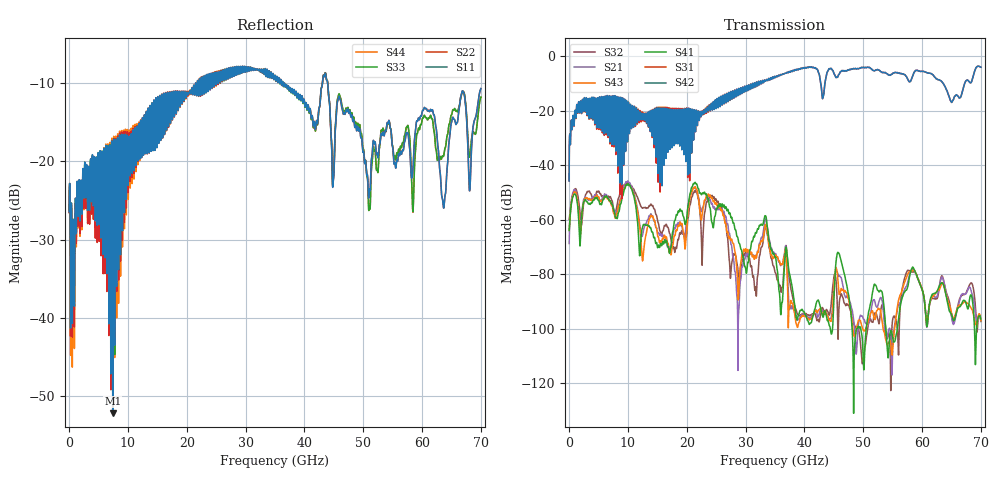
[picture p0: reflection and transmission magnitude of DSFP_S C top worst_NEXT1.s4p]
! AWR Design Environment (8415) Wed Jan 09 11:08:23 2019
! Document = 'DSFP_S'
! nPorts: 4, nXvals: 7001
# HZ S DB R 50
!Freq DBS11 AngS11 DBS12 AngS12 DBS13 AngS13 DBS14 AngS14
!	DBS21 AngS21 DBS22 AngS22 DBS23 AngS23 DBS24 AngS24
!	DBS31 AngS31 DBS32 AngS32 DBS33 AngS33 DBS34 AngS34
!	DBS41 AngS41 DBS42 AngS42 DBS43 AngS43 DBS44 AngS44
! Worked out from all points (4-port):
!   7000 points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, 10 MHz to 70 GHz, reference 50 ohm
!   strongest paths, dB at 10 MHz, 17.51 GHz, 35.01 GHz, 52.51 GHz, 70 GHz:
!     S42: -45.8, -29.4, -7.6, -5.0, -4.0
!     S31: -45.8, -28.1, -7.6, -5.0, -4.0
!     S41: -64.0, -66.0, -73.7, -86.0, -96.5
!     S43: -63.7, -70.0, -73.7, -92.7, -97.0
!     S21: -68.8, -66.5, -72.7, -91.4, -97.0
!     S32: -59.8, -68.3, -79.3, -96.8, -97.4
!   lowest |S11| = -52.2 dB at 7.42 GHz (marker M1), VSWR 1.00, Z = 50 + j0.24 ohm
!   |S11| at or under -10 dB: start of sweep to 21.5 GHz; 36.64 GHz to 43.07 GHz (6.432 GHz wide, 16.1 % of centre); 43.96 GHz to end of sweep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
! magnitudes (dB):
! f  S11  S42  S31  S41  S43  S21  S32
! 10 MHz  -26.4  -45.8  -45.8  -64.0  -63.7  -68.8  -59.8
! 7.42 GHz  -52.2  -15.2  -15.4  -55.0  -55.9  -55.0  -54.2
! 17.05 GHz  -11.2  -21.9  -21.3  -72.4  -72.0  -72.1  -64.9
! 21.41 GHz  -11.1  -22.3  -22.4  -46.3  -47.9  -48.0  -49.3
! 28.63 GHz  -8.6  -13.7  -13.8  -66.3  -82.1  -92.6  -77.0
! 33.43 GHz  -8.6  -9.1  -9.1  -58.7  -61.8  -59.8  -62.7
! 70 GHz  -10.7  -4.0  -4.0  -96.5  -97.0  -97.0  -97.4
